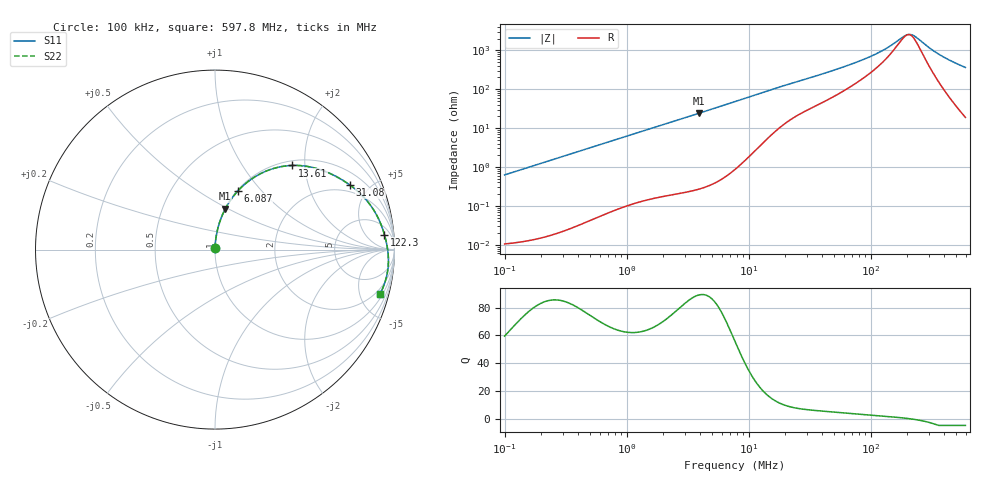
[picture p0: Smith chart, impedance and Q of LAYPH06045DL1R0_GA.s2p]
! LAYPH06045DL1R0_GA  S-PARAMETER MODEL  ( General Type )
! Model Generated by TAIYO YUDEN Corporation (http://www.ty-top.com)
! Version 2.0
! TAIYO YUDEN Control No. 180914NI43SB-FBB
! Copyright(c) 2018 TAIYO YUDEN CO.,LTD. All Rights Reserved.
! Product Description (link to TY-COMPAS)
! https://ds.yuden.co.jp/TYCOMPAS/or/detail?pn=LAYPH06045DL1R0NGA&u=M
! Products Name : Inductors
! Characteristics :
!  Inductance : 1.0 uH , SRF(min) : -Hz , DC Resistance(max) : 0.0117 Ohm
!  Rated Current : Saturation :6.7 A , Temp Rise : 3.5 A (25 degC)
!  Case Size : 6.3 x 6.0 / 0.248 x 0.236 [mm/inch] , Thickness : 4.5 / 0.177 [mm/inch]
!  (Conditions: Temperature = 25 degC , DC Bias Current/Voltage = 0A / 0V)
! External Node Assignments :
!  1  o---GGG---o  2
! GND o---------o GND
! Frequency Range : 0.1MHz  -  597.797849MHz  [ 402 STEP ]
# MHz S RI R 50
! Freq[MHz].  S11 Real  S11 Imag  S21 Real  S21 Imag  S12 Real  S12 Imag  S22 Real  S22 Imag
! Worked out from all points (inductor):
!   401 points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, 100 kHz to 597.8 MHz, reference 50 ohm
!   read as one part in series: L = 997 nH near 104.4 kHz
!   highest Q = 89.2 at 3.941 MHz (marker M1), where L = 977 nH
!   self-resonance near 202.1 MHz
!   S11 on the Smith chart (normalised r, x): 100 kHz: 1.00, +0.01; 6.087 MHz: 1.01, +0.75; 13.61 MHz: 1.09, +1.72; 31.08 MHz: 1.61, +3.79; 122.3 MHz: 10, +17; 597.8 MHz: 1.38, -7.24
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0.1  0.000145 0.00626  0.9999 -0.00626  0.9999 -0.00626  0.000145 0.00626
0.429114  0.00106 0.0268  0.9989 -0.0268  0.9989 -0.0268  0.00106 0.0268
1.84139  0.0143 0.1114  0.9857 -0.1114  0.9857 -0.1114  0.0143 0.1114
3.940889  0.0576 0.2274  0.9424 -0.2274  0.9424 -0.2274  0.0576 0.2274
6.087261  0.1272 0.3266  0.8728 -0.3266  0.8728 -0.3266  0.1272 0.3266
7.731739  0.1921 0.385  0.8079 -0.385  0.8079 -0.385  0.1921 0.385
13.60671  0.4309 0.4689  0.5691 -0.4689  0.5691 -0.4689  0.4309 0.4689
20.56551  0.6165 0.4345  0.3835 -0.4345  0.3835 -0.4345  0.6165 0.4345
31.08321  0.7538 0.3583  0.2462 -0.3583  0.2462 -0.3583  0.7538 0.3583
33.17799  0.7716 0.3448  0.2284 -0.3448  0.2284 -0.3448  0.7716 0.3448
69.47957  0.904 0.1858  0.096 -0.1858  0.096 -0.1858  0.904 0.1858
94.19689  0.9294 0.128  0.0706 -0.128  0.0706 -0.128  0.9294 0.128
122.2737  0.9441 0.0832  0.0559 -0.0832  0.0559 -0.0832  0.9441 0.0832
142.3714  0.9507 0.0582  0.0493 -0.0582  0.0493 -0.0582  0.9507 0.0582
188.8691  0.9602 0.0116  0.0398 -0.0116  0.0398 -0.0116  0.9602 0.0116
201.5975  0.9619 0.000477  0.0381 -0.000477  0.0381 -0.000477  0.9619 0.000477
215.1836  0.9634 -0.0109  0.0366 0.0109  0.0366 0.0109  0.9634 -0.0109
234.7333  0.9649 -0.0266  0.0351 0.0266  0.0351 0.0266  0.9649 -0.0266
304.6993  0.966 -0.0781  0.034 0.0781  0.034 0.0781  0.966 -0.0781
370.5475  0.9615 -0.122  0.0385 0.122  0.0385 0.122  0.9615 -0.122
470.6511  0.9468 -0.1824  0.0532 0.1824  0.0532 0.1824  0.9468 -0.1824
597.7978  0.918 -0.2495  0.082 0.2495  0.082 0.2495  0.918 -0.2495
